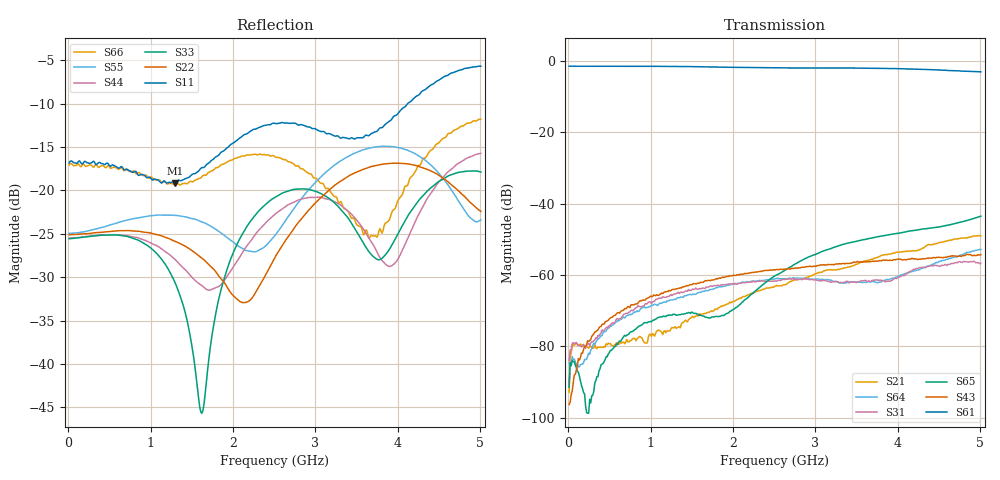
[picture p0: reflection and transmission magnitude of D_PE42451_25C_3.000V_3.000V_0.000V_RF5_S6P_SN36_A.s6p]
! Device ID: PE42451
! Serial: 36
! Insertion: A
! Temp: 25C
! VDD: 3.000
! Control_Hi: 100.000
! Control_Lo: 0.000
! Logic State: RF5
! Port 1: RFC
! Port 2: RF1
! Port 3: RF2
! Port 4: RF3
! Port 5: RF4
! Port 6: RF5
! V1 = 3.00
! V2 = 0.00
! V3 = 3.00
! V4 = 0.00
! IDD: 1.335240e-05
#  Hz  S  RI  R  50
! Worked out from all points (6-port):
!   401 points, 10 MHz to 5.01 GHz, reference 50 ohm
!   strongest paths, dB at 10 MHz, 1.26 GHz, 2.51 GHz, 3.76 GHz, 5.01 GHz:
!     S61: -1.5, -1.6, -2.0, -2.1, -3.1
!     S43: -96.3, -64.1, -58.6, -56.1, -54.3
!     S65: -91.4, -71.3, -60.2, -49.3, -43.5
!     S31: -83.9, -65.8, -61.7, -61.5, -56.6
!     S64: -84.5, -67.0, -61.0, -62.2, -52.9
!     S21: -92.9, -74.6, -63.1, -55.0, -49.1
!   lowest |S11| = -19.2 dB at 1.298 GHz (marker M1), VSWR 1.25, Z = 54.6 - j10.6 ohm
!   |S11| at or under -10 dB: start of sweep to 4.118 GHz
